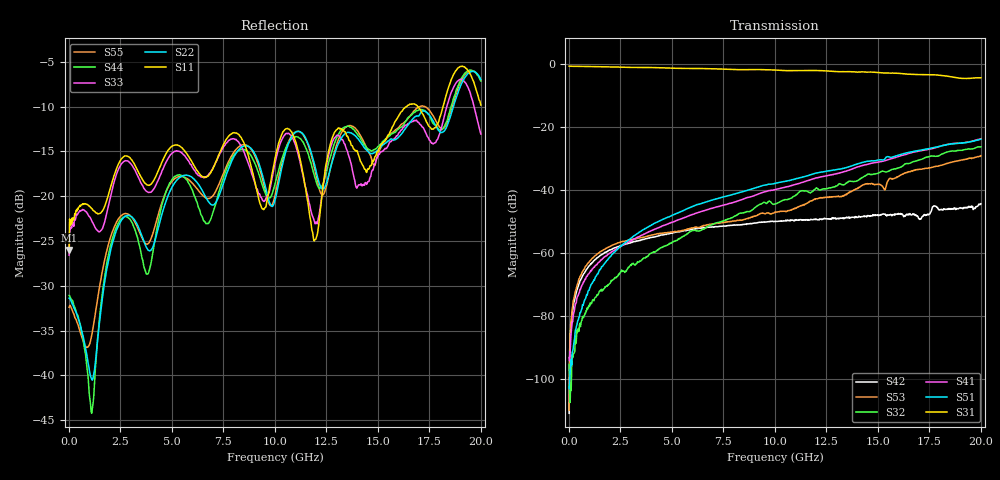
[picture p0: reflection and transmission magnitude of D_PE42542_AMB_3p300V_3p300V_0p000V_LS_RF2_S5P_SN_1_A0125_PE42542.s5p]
! Device ID: PE42542
! Device ID: PE42542
! File Path: z:\PE42542\PE42543_20140723_inv\AMB\3p300\LS_RF2\PE42542_AMB_3p300V_3p300V_0p000V_LS_RF2_S5P_SN_1_A0125_PE42542.s5p
! Serial: 1
! Lot: A0125_PE42542
! Temp: AMB
! VDD: 3.300
! VSS: 0.000
! Control_Hi: 3.300
! Control_Lo: 0.000
! Logic State: LS_RF2
! Port 1: RFC
! Port 2: RF1
! Port 3: RF2
! Port 5: RF3
! Port 6: RF4
! ThroughPath:1-3
! IDD: -0.000143285769
! ISS: -8.65565341e-010
#  Hz  S  RI  R  50
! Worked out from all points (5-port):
!   801 points, 10 MHz to 20 GHz, reference 50 ohm
!   strongest paths, dB at 10 MHz, 5.008 GHz, 10.01 GHz, 15 GHz, 20 GHz:
!     S31: -0.7, -1.3, -1.9, -2.7, -4.4
!     S51: -103.0, -48.0, -37.9, -30.5, -23.8
!     S41: -93.1, -50.2, -39.8, -31.2, -23.7
!     S32: -95.3, -56.6, -44.4, -34.7, -26.3
!     S53: -109.8, -53.3, -46.9, -38.1, -29.1
!     S42: -110.8, -53.7, -49.9, -47.8, -44.4
!   lowest |S11| = -26.0 dB at 10 MHz (marker M1), VSWR 1.11, Z = 54.7 - j2.31 ohm
!   |S11| at or under -10 dB: start of sweep to 16.37 GHz; 16.94 GHz to 18.16 GHz (1.221 GHz wide, 6.96 % of centre)
